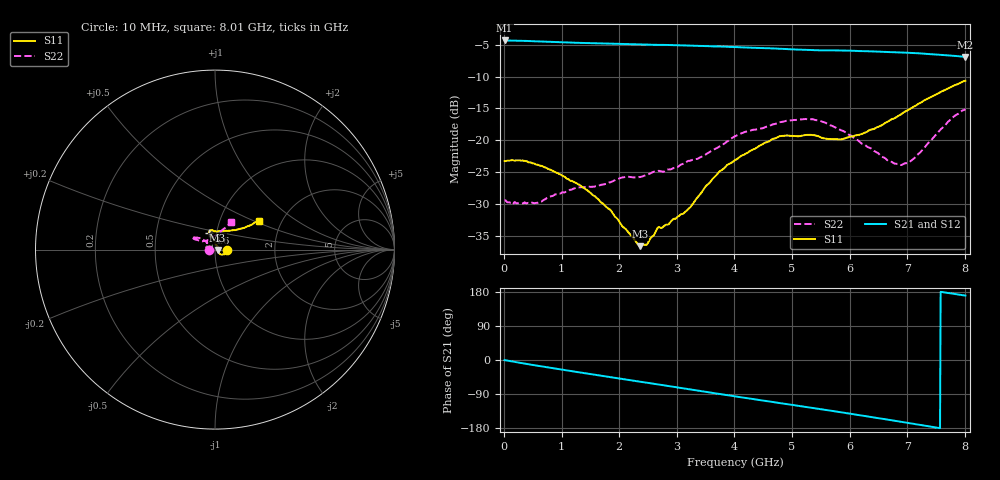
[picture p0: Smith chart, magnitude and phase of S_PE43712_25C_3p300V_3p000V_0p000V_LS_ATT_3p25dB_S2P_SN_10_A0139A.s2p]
! DEVICE ID: PE43712
! File Path: z:\PE43713\PE43713_CHAR_NOM_04292014\AMB\3p300\LS_ATT_3p25dB\PE43713_AMB_3p300V_3p000V_0p000V_LS_ATT_3p25dB_S2P_SN_10_A0139A.s2p
! Serial: 10
! Lot: A0139A
! Temp: 25C
! VDD: 3.300
! VSS: 0.000
! Control_Hi: 3.000
! Control_Lo: 0.000
! Attenuation Step: 3.25dB
! Port 1: RF1
! Port 2: RF2
! ThroughPath:1-2
! IDD: 0.0001470883
! ISS: -1.694e-007
#  Hz  S  RI  R  50
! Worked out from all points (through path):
!   801 points, 10 MHz to 8.01 GHz, reference 50 ohm
!   highest |S21| = -4.33 dB at 10 MHz (marker M1); lowest = -6.9 dB at 8.01 GHz (marker M2)
!   group delay of S21, straight-line fit = 65.1 ps
!   lowest |S11| = -36.7 dB at 2.36 GHz (marker M3), VSWR 1.03, Z = 51.5 - j0.229 ohm
!   |S11| at or under -10 dB: start of sweep to end of sweep
!   |S22| runs from -30.1 to -15.1 dB; largest |S21 - S12| = 0.0017
!   S11 on the Smith chart (normalised r, x): 10 MHz: 1.15, -0.00; 4.6 GHz: 0.92, +0.17; 8.01 GHz: 1.53, +0.54
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1e7  0.0685 -0.000354  0.6078 -0.00333  0.6077 -0.00315  -0.0337 5.69e-05
3e8  0.0678 -0.0134  0.5977 -0.0843  0.5971 -0.0843  -0.0319 -0.00222
5.6e8  0.0607 -0.0213  0.5786 -0.1511  0.5783 -0.1511  -0.0319 -0.00382
1.35e9  0.0333 -0.0273  0.4841 -0.3218  0.4841 -0.3218  -0.0427 -0.00118
1.85e9  0.0217 -0.018  0.4037 -0.4073  0.4037 -0.4072  -0.0458 0.00913
2.08e9  0.0162 -0.0128  0.3617 -0.4411  0.3617 -0.4408  -0.0492 0.0139
2.36e9  0.0145 -0.00223  0.3064 -0.4762  0.3065 -0.4761  -0.0463 0.0222
2.48e9  0.015 0.0024  0.2816 -0.4889  0.2817 -0.4888  -0.0458 0.0282
2.68e9  0.0163 0.0128  0.2408 -0.5064  0.2409 -0.5064  -0.042 0.0392
3.15e9  0.00603 0.0268  0.1369 -0.538  0.137 -0.538  -0.0501 0.044
3.71e9  -0.00505 0.0544  0.0116 -0.5446  0.0114 -0.5448  -0.0669 0.0564
4.01e9  -0.0161 0.0678  -0.0554 -0.537  -0.0552 -0.5369  -0.086 0.0641
4.6e9  -0.0327 0.0923  -0.1768 -0.4977  -0.1765 -0.4978  -0.1107 0.0668
4.81e9  -0.0311 0.1033  -0.2167 -0.4759  -0.2162 -0.4762  -0.1209 0.0684
5.35e9  -0.0191 0.1081  -0.3044 -0.4105  -0.3043 -0.4101  -0.1299 0.0671
5.87e9  0.0112 0.1011  -0.3794 -0.3361  -0.3785 -0.3362  -0.1049 0.0558
6.24e9  0.0466 0.1035  -0.421 -0.2714  -0.4199 -0.2711  -0.0802 0.047
6.68e9  0.0931 0.1067  -0.4562 -0.1857  -0.4559 -0.1856  -0.047 0.0494
6.89e9  0.1162 0.1089  -0.4676 -0.1429  -0.4671 -0.1429  -0.0292 0.0567
7.05e9  0.1345 0.1143  -0.4731 -0.1094  -0.4726 -0.1094  -0.0133 0.0666
7.72e9  0.2123 0.1444  -0.4624 0.0285  -0.4622 0.028  0.0621 0.1266
8.01e9  0.2449 0.1617  -0.4448 0.0788  -0.4436 0.078  0.0885 0.1512
